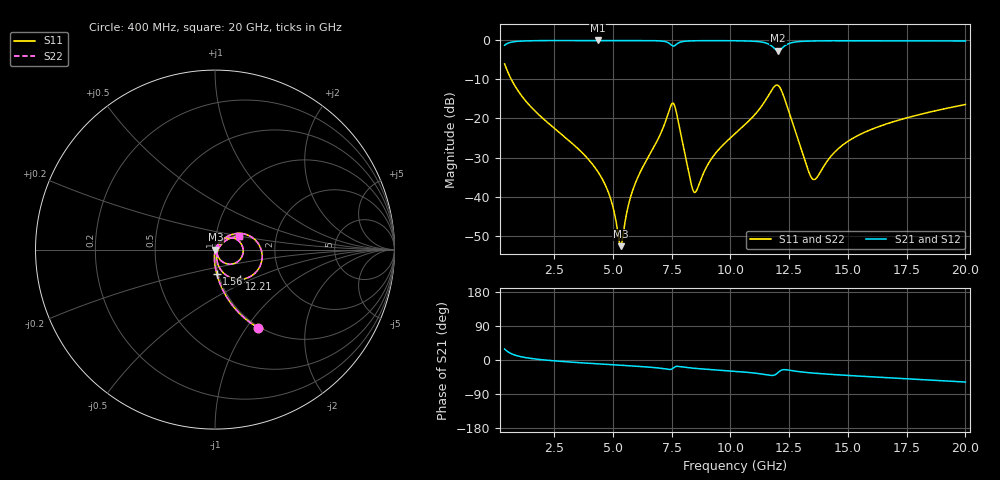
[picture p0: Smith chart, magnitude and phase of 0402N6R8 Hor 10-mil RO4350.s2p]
# MHz S  dB  R 50
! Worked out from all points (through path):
!   1961 points, 400 MHz to 20 GHz, reference 50 ohm
!   highest |S21| = -0.02 dB at 4.37 GHz (marker M1); lowest = -2.7 dB at 12.03 GHz (marker M2)
!   group delay of S21, straight-line fit = 8.95 ps
!   lowest |S11| = -52.7 dB at 5.34 GHz (marker M3), VSWR 1.00, Z = 50.2 - j0.0546 ohm
!   |S11| at or under -10 dB: 685.8 MHz to end of sweep
!   |S22| runs from -52.7 to -6.0 dB; largest |S21 - S12| = 0
!   S11 on the Smith chart (normalised r, x): 400 MHz: 0.98, -1.14; 1.56 GHz: 0.98, -0.27; 12.21 GHz: 1.24, -0.43; 20 GHz: 1.28, +0.20
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400  -6.03 -61.0  -1.25 28.9  -1.25 28.9  -6.03 -61.0
800  -11.26 -76.1  -0.34 13.8  -0.34 13.8  -11.26 -76.1
1560  -17.27 -85.8  -0.09 3.8  -0.09 3.8  -17.27 -85.8
3670  -28.59 -94.9  -0.02 -7.4  -0.02 -7.4  -28.59 -94.9
4370  -33.65 -95.1  -0.02 -10.2  -0.02 -10.2  -33.65 -95.1
4900  -40.37 -89.8  -0.02 -12.2  -0.02 -12.2  -40.37 -89.8
5340  -52.69 -13.5  -0.02 -13.8  -0.02 -13.8  -52.69 -13.5
5890  -37.68 61.0  -0.03 -16.0  -0.03 -16.0  -37.68 61.0
6940  -25.11 57.2  -0.12 -21.1  -0.12 -21.1  -25.11 57.2
7600  -16.29 -17.4  -1.45 -20.0  -1.45 -20.0  -16.29 -17.4
8330  -36.59 -43.6  -0.12 -21.1  -0.12 -21.1  -36.59 -43.6
8500  -38.93 -4.0  -0.10 -22.1  -0.10 -22.1  -38.93 -4.0
9210  -30.21 51.5  -0.07 -25.4  -0.07 -25.4  -30.21 51.5
10200  -23.90 52.6  -0.10 -29.8  -0.10 -29.8  -23.90 52.6
11580  -14.55 27.4  -0.81 -39.5  -0.81 -39.5  -14.55 27.4
12030  -11.53 -23.8  -2.65 -33.2  -2.65 -33.2  -11.53 -23.8
12210  -13.33 -50.4  -1.95 -26.0  -1.95 -26.0  -13.33 -50.4
12590  -20.03 -76.8  -0.62 -27.7  -0.62 -27.7  -20.03 -76.8
13470  -35.29 -33.9  -0.16 -34.2  -0.16 -34.2  -35.29 -33.9
14890  -26.31 39.8  -0.09 -40.3  -0.09 -40.3  -26.31 39.8
16740  -21.20 39.0  -0.09 -46.9  -0.09 -46.9  -21.20 39.0
20000  -16.42 29.8  -0.16 -58.1  -0.16 -58.1  -16.42 29.8
